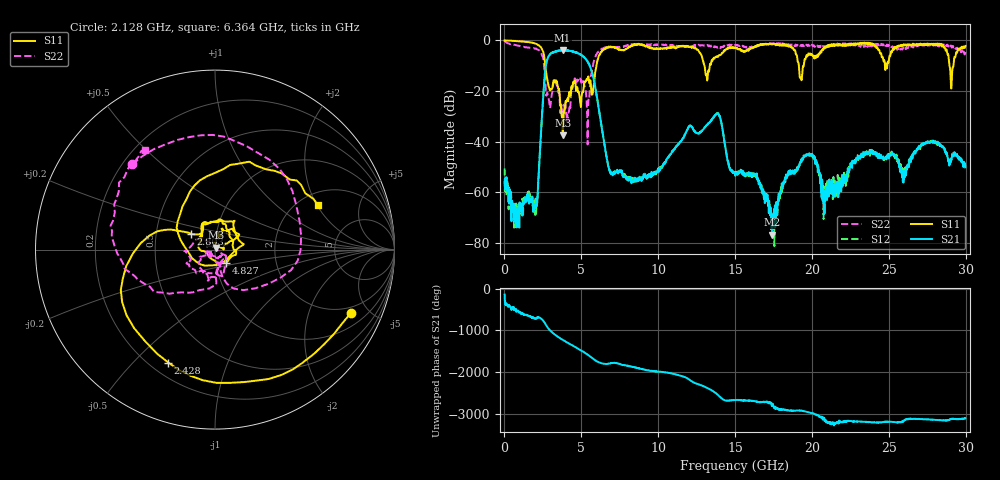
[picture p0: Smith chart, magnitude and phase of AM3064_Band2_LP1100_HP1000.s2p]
# Hz S DB R 50.0
!freq dBS11 angS11 dBS21 angS21 dBS12 angS12 dBS22 angS22
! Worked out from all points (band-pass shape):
!   1600 points, 10 MHz to 29.98 GHz, reference 50 ohm
!   highest |S21| = -3.84 dB at 3.777 GHz (marker M1); lowest = -76.7 dB at 17.4 GHz (marker M2)
!   |S21| within 3 dB of the highest: 2.829 GHz to 5.197 GHz (2.368 GHz wide, 59 % of centre)
!   lowest |S11| = -37.4 dB at 3.796 GHz (marker M3), VSWR 1.03, Z = 50.8 + j1.11 ohm
!   |S11| at or under -10 dB: 2.663 GHz to 5.984 GHz (3.321 GHz wide, 76.8 % of centre); 13.01 GHz to 13.35 GHz (337.5 MHz wide, 2.56 % of centre); 19.15 GHz to 19.46 GHz (312.9 MHz wide, 1.62 % of centre)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
!   |S22| runs from -41.1 to -0.3 dB; largest |S21 - S12| = 0.023
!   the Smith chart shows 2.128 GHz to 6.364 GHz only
!   S11 on the Smith chart (normalised r, x): 2.128 GHz: 1.66, -3.87; 2.428 GHz: 0.27, -0.63; 2.803 GHz: 0.75, +0.14; 4.827 GHz: 1.12, -0.16; 6.364 GHz: 2.49, +2.03
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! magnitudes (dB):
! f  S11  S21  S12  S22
! 10 MHz  -0.1  -55.9  -50.6  -0.3
! 722.3 MHz  -0.2  -72.5  -74.5  -1.9
! 2.128 GHz  -1.6  -64.2  -63.0  -3.6
! 2.428 GHz  -3.3  -31.0  -31.1  -5.7
! 2.803 GHz  -15.8  -7.2  -7.1  -21.1
! 3.777 GHz  -35.4  -3.8  -4.0  -30.5
! 3.796 GHz  -37.4  -3.9  -3.9  -28.5
! 4.827 GHz  -20.3  -5.2  -5.2  -15.2
! 5.015 GHz  -22.3  -5.8  -5.8  -16.6
! 5.408 GHz  -14.9  -8.3  -8.3  -41.1
! 6.364 GHz  -4.1  -35.8  -35.8  -3.3
! 6.964 GHz  -2.6  -52.5  -52.9  -2.7
! 10 GHz  -3.4  -51.0  -50.0  -1.8
! 13.84 GHz  -6.3  -28.9  -28.9  -2.9
! 15 GHz  -2.8  -53.5  -53.1  -1.8
! 16.39 GHz  -2.2  -54.2  -54.0  -2.6
! 17.4 GHz  -1.6  -76.7  -72.9  -1.3
! 19.99 GHz  -5.4  -45.5  -45.2  -1.7
! 20.83 GHz  -3.2  -63.3  -59.9  -2.3
! 25 GHz  -8.3  -46.6  -44.9  -1.8
! 29.08 GHz  -17.7  -46.3  -47.3  -2.7
! 29.98 GHz  -2.2  -49.9  -50.5  -4.7
